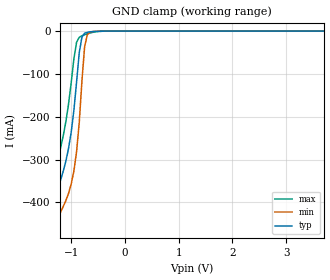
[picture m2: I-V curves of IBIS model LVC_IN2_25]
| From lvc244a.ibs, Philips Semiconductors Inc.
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|   Model LVC_IN2_25
[Model]   LVC_IN2_25
Model_type   Input
Vinl =   0.7000V
Vinh =   1.7000V
C_comp   2.84pF   2.10pF   3.71pF
[Model Spec]
| Note: The input and output voltage ratings may be exceeded if the input and
|   output current ratings are observed (please refer to the data sheet)
|   Subparameter   typ   min   max
| Thresholds
Vinh   1.7   NA   NA
Vinl   0.7   NA   NA
| Overshoot
S_overshoot_high   6.5   6.5   6.5   | Static overshoot
S_overshoot_low   -0.5   -0.5   -0.5
D_overshoot_high   7.2   7.2   7.2   | Dynamic overshoot
D_overshoot_low   -0.95   -0.9   -1.0
D_overshoot_time   3n   3n   3n
|Ambient temperature:   25.0000   85.0000   -40.0000
[Temperature Range]   35.0000   95.0000   -30.0000
[Voltage Range]   2.5000V   2.3000V   2.7000V
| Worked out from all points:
|   GND clamp passes 1 mA (typ) near -0.57 V on its own axis
|Process Range   nominal   slow   fast
[GND_clamp]
| voltage   I(typ)   I(min)   I(max)
-5.5V     -4.558A    -4.615A    -4.502A
-1.45V    -549mA     -615mA     -482.5mA
-1.35V    -455.6mA   -522.2mA   -388.4mA
-1.3V     -411.3mA   -478.6mA   -343.5mA
-1.1V     -304mA     -396mA     -212mA
-950mV    -185.1mA   -326.6mA   -65.02mA
-900mV    -119.1mA   -281.8mA   -26.08mA
-850mV    -50.24mA   -213.2mA   -14.46mA
-800mV    -13.81mA   -116mA     -10.88mA
-750mV    -4.865mA   -35.92mA   -8.446mA
-700mV    -2.732mA   -8.828mA   -6.333mA
5.5V      922.9pA    6.4nA      86.94pA
